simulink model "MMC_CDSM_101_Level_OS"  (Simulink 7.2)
settings: Solver=ode3  StartTime=0.0  StopTime=0.25  FixedStep=4e-6  MaxStep=5e-5  RelTol=1e-3  AbsTol=1e-3
PreLoadFcn:
  | INIT_MMC_100L
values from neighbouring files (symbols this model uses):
  C = 5e-3*1    (= 0.005)    [INIT_MMC_100L.m]    (also in INIT_MMC_200L.m; INIT_MMC_20L.m = 0.01; INIT_MMC_400L.m = 0.01; INIT_B6_2L_3Ph_IGBT_OS.m = 0.01)
  F = 50    [INIT_MMC_100L.m]    (also in INIT_MMC_200L.m; INIT_MMC_20L.m; INIT_MMC_400L.m; INIT_B6_2L_3Ph_IGBT_OS.m)
  FS = 50    [INIT_MMC_100L.m]    (also in INIT_MMC_200L.m; INIT_MMC_20L.m = 150; INIT_MMC_400L.m; INIT_B6_2L_3Ph_IGBT_OS.m = 900)
  I_B = INS    [INIT_MMC_100L.m]    (also in INIT_MMC_200L.m; INIT_MMC_20L.m; INIT_MMC_400L.m; INIT_B6_2L_3Ph_IGBT_OS.m)
  IDC = PDC/VDC    (= 1562.5)    [INIT_MMC_100L.m]    (also in INIT_MMC_200L.m; INIT_MMC_20L.m = 1000; INIT_MMC_400L.m; INIT_B6_2L_3Ph_IGBT_OS.m = 166.666666667)
  KI2 = 0.01    [INIT_MMC_100L.m]    (also in INIT_MMC_200L.m = 100; INIT_MMC_20L.m = 0.1; INIT_MMC_400L.m = 0.1)
  KP2 = 0.2    [INIT_MMC_100L.m]    (also in INIT_MMC_200L.m; INIT_MMC_20L.m = 1; INIT_MMC_400L.m)
  LN = 25e-3    (= 0.025)    [INIT_MMC_100L.m]    (also in INIT_MMC_200L.m; INIT_MMC_20L.m = 0.002; INIT_MMC_400L.m; INIT_PWM_2L.m = 0.002)
  LNpu = LN/L_B    [INIT_MMC_100L.m]    (also in INIT_MMC_200L.m; INIT_MMC_20L.m; INIT_MMC_400L.m; INIT_PWM_2L.m)
  LS = 25e-3    (= 0.025)    [INIT_MMC_100L.m]    (also in INIT_MMC_200L.m; INIT_MMC_20L.m = 0.0025; INIT_MMC_400L.m; INIT_B6_2L_3Ph_IGBT_OS.m = 0.001)
  LSpu = LS/L_B    [INIT_MMC_100L.m]    (also in INIT_MMC_200L.m; INIT_MMC_20L.m; INIT_MMC_400L.m; INIT_B6_2L_3Ph_IGBT_OS.m)
  LT = LN    (= 0.025)    [INIT_MMC_100L.m]    (also in INIT_MMC_200L.m; INIT_MMC_20L.m = 0.002; INIT_MMC_400L.m)
  Nc = 100    [INIT_MMC_100L.m]    (also in INIT_MMC_200L.m = 200; INIT_MMC_20L.m = 20; INIT_MMC_400L.m = 400)
  NT = sqrt(3)*340/400    [INIT_MMC_100L.m]    (also in INIT_MMC_200L.m; INIT_MMC_20L.m = sqrt(3); INIT_MMC_400L.m)
  RN = 0.1    [INIT_MMC_100L.m]    (also in INIT_MMC_200L.m; INIT_MMC_20L.m; INIT_MMC_400L.m; INIT_PWM_2L.m)
  RT = RN    (= 0.1)    [INIT_MMC_100L.m]    (also in INIT_MMC_200L.m; INIT_MMC_20L.m; INIT_MMC_400L.m)
  U_B = UNS    [INIT_MMC_100L.m]    (also in INIT_MMC_200L.m; INIT_MMC_20L.m; INIT_MMC_400L.m; INIT_B6_2L_3Ph_IGBT_OS.m)
  UC0 = 3.4e3*2    (= 6800)    [INIT_MMC_100L.m]    (also in INIT_MMC_200L.m = 3400; INIT_MMC_20L.m = 5000; INIT_MMC_400L.m = 1700; INIT_B6_2L_3Ph_IGBT_OS.m = 600)
  UNP = ULLP/sqrt(3)    [INIT_MMC_100L.m]    (also in INIT_MMC_200L.m; INIT_MMC_20L.m; INIT_MMC_400L.m; INIT_B6_2L_3Ph_IGBT_OS.m)
  UNS = ULLP/sqrt(3)*340/400    [INIT_MMC_100L.m]    (also in INIT_MMC_200L.m; INIT_MMC_20L.m = ULLP/sqrt(3); INIT_MMC_400L.m; INIT_B6_2L_3Ph_IGBT_OS.m = ULLP/sqrt(3))
  VDC = 640e3    (= 640000)    [INIT_MMC_100L.m]    (also in INIT_MMC_200L.m; INIT_MMC_20L.m = 100000; INIT_MMC_400L.m; INIT_B6_2L_3Ph_IGBT_OS.m = 600)
libraries: simulink x1

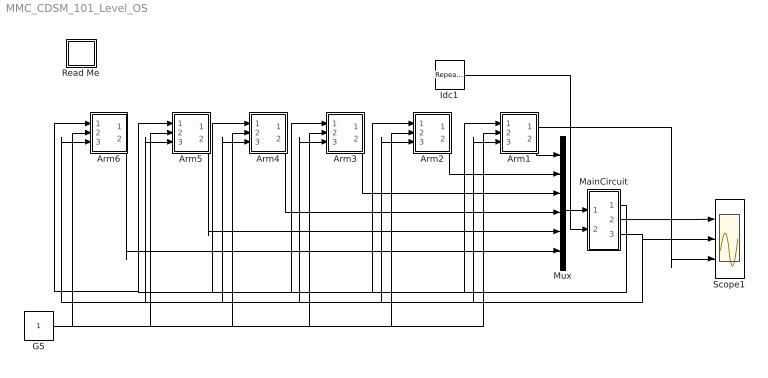
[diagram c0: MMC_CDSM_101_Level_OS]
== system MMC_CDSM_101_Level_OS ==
  Arm1 : Subsystem
  Arm2 : Subsystem
  Arm3 : Subsystem
  Arm4 : Subsystem
  Arm5 : Subsystem
  Arm6 : Subsystem
  G5 : Constant  OutDataType=sfix(16)  OutScaling=2^0
  Idc1 : simulink/Sources/Repeating Sequence  SystemSampleTime=-1  rep_seq_t="[0    0.1   0.101   0.15    0.151   5 ]"  rep_seq_y="[1     1       0.0        0.0       -1         -1 ]*IDC"
  MainCircuit : Subsystem
  Mux : Mux  Inputs=6
  Read Me : Subsystem
  Scope1 : Scope  NumInputPorts=3
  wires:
  Mux/1 -> MainCircuit/1(V)
  MainCircuit/1(G) -> Arm1/1(G1), Arm5/1(G1), Arm6/1(G1), Arm4/1(G1), Arm3/1(G1), Arm2/1(G1)
  MainCircuit/3(ILs) -> Arm1/3(ILs), Arm5/3(ILs), Arm6/3(ILs), Arm4/3(ILs), Arm3/3(ILs), Arm2/3(ILs), Scope1/2
  Idc1/1 -> MainCircuit/2(Idc)
  MainCircuit/2(IWR) -> Scope1/1
  Arm1/1(VC) -> Scope1/3
  Arm1/2(V1) -> Mux/1
  Arm2/2(V1) -> Mux/2
  Arm3/2(V1) -> Mux/3
  Arm4/2(V1) -> Mux/4
  Arm5/2(V1) -> Mux/5
  Arm6/2(V1) -> Mux/6
  G5/1 -> Arm1/2(G5), Arm2/2(G5), Arm3/2(G5), Arm4/2(G5), Arm5/2(G5), Arm6/2(G5)

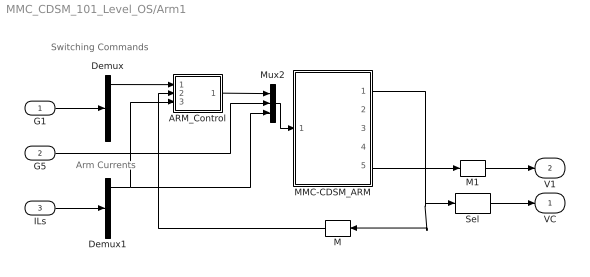
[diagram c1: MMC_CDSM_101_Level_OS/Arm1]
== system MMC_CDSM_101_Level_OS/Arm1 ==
  note: Switching Commands
  note: Arm Currents
  G1 : Inport
  G5 : Inport  Port=2
  ILs : Inport  Port=3
  ARM_Control : Subsystem
  Demux : Demux  Outputs=6
  Demux1 : Demux  Outputs=6
  M : Memory  Orientation=left
  M1 : Memory
  MMC-CDSM_ARM : Subsystem  mask(MMC_HB_ARM){C=C, UC0=UC0, Nc=Nc}
      mask prompts: C "C [F]"; UC0 "UC0 [V]"; Nc "Number Caps"
      mask help: Input Vector Switching Signals Arm Current Output Vector Capacitor Voltages Capacitor Current IT1, ID1, VT1, IT2, ID2, VT2 Arm Voltage Parameter Vector Capacitor Value =p[0] Initial Capacitor Voltage =p[1] Number of Cap. =p[2]
  Mux2 : Mux  Inputs="[2*Nc  1  1]"
  Sel : Selector  InputPortWidth=Nc  IndexOptions=Index vector (dialog)  Indices=[1 2 3 4 5 6 7 8 9 10]  OutputSizes=1
  VC : Outport
  V1 : Outport  Port=2
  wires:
  ARM_Control/1(O1) -> Mux2/1
  ILs/1 -> Demux1/1
  MMC-CDSM_ARM/1(VCs) -> M/1, Sel/1
  M/1 -> ARM_Control/2(Uc)
  Demux1/1 -> ARM_Control/3(ILs), Mux2/3
  G1/1 -> Demux/1
  Demux/1 -> ARM_Control/1(S)
  Mux2/1 -> MMC-CDSM_ARM/1(In)
  MMC-CDSM_ARM/5(V_arm) -> M1/1
  M1/1 -> V1/1
  Sel/1 -> VC/1
  G5/1 -> Mux2/2

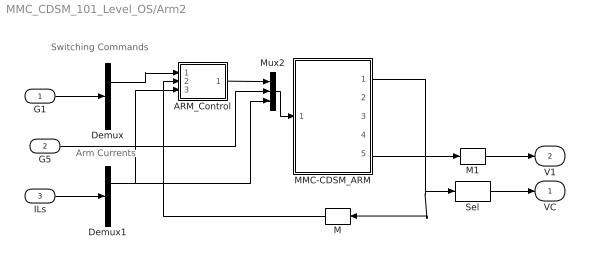
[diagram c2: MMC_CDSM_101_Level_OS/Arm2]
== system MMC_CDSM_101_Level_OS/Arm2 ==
  note: Arm Currents
  note: Switching Commands
  G1 : Inport
  G5 : Inport  Port=2
  ILs : Inport  Port=3
  ARM_Control : Subsystem
  Demux : Demux  Outputs=6
  Demux1 : Demux  Outputs=6
  M : Memory  Orientation=left
  M1 : Memory
  MMC-CDSM_ARM : Subsystem  mask(MMC_HB_ARM){C=C, UC0=UC0, Nc=Nc}
      mask prompts: C "C [F]"; UC0 "UC0 [V]"; Nc "Number Caps"
      mask help: Input Vector Switching Signals Arm Current Output Vector Capacitor Voltages Capacitor Current IT1, ID1, VT1, IT2, ID2, VT2 Arm Voltage Parameter Vector Capacitor Value =p[0] Initial Capacitor Voltage =p[1] Number of Cap. =p[2]
  Mux2 : Mux  Inputs="[2*Nc 1  1]"
  Sel : Selector  InputPortWidth=Nc  IndexOptions=Index vector (dialog)  Indices=[1 2 3 4 5 6 7 8 9 10]  OutputSizes=1
  VC : Outport
  V1 : Outport  Port=2
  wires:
  Sel/1 -> VC/1
  M1/1 -> V1/1
  MMC-CDSM_ARM/5(V_arm) -> M1/1
  Mux2/1 -> MMC-CDSM_ARM/1(In)
  G1/1 -> Demux/1
  M/1 -> ARM_Control/2(Uc)
  MMC-CDSM_ARM/1(VCs) -> Sel/1, M/1
  ILs/1 -> Demux1/1
  ARM_Control/1(O1) -> Mux2/1
  Demux1/2 -> ARM_Control/3(ILs), Mux2/3
  Demux/2 -> ARM_Control/1(S)
  G5/1 -> Mux2/2

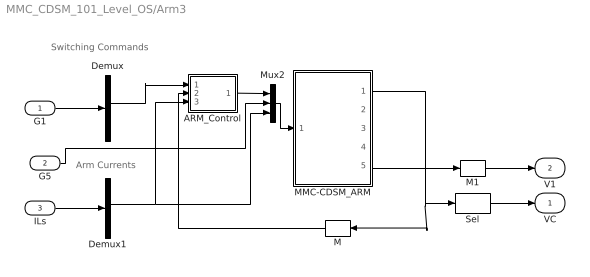
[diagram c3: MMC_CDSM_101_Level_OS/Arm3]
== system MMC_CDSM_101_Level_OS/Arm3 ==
  note: Switching Commands
  note: Arm Currents
  G1 : Inport
  G5 : Inport  Port=2
  ILs : Inport  Port=3
  ARM_Control : Subsystem
  Demux : Demux  Outputs=6
  Demux1 : Demux  Outputs=6
  M : Memory  Orientation=left
  M1 : Memory
  MMC-CDSM_ARM : Subsystem  mask(MMC_HB_ARM){C=C, UC0=UC0, Nc=Nc}
      mask prompts: C "C [F]"; UC0 "UC0 [V]"; Nc "Number Caps"
      mask help: Input Vector Switching Signals Arm Current Output Vector Capacitor Voltages Capacitor Current IT1, ID1, VT1, IT2, ID2, VT2 Arm Voltage Parameter Vector Capacitor Value =p[0] Initial Capacitor Voltage =p[1] Number of Cap. =p[2]
  Mux2 : Mux  Inputs="[2*Nc  1  1]"
  Sel : Selector  InputPortWidth=Nc  IndexOptions=Index vector (dialog)  Indices=[1 2 3 4 5 6 7 8 9 10]  OutputSizes=1
  VC : Outport
  V1 : Outport  Port=2
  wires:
  ARM_Control/1(O1) -> Mux2/1
  ILs/1 -> Demux1/1
  MMC-CDSM_ARM/1(VCs) -> M/1, Sel/1
  M/1 -> ARM_Control/2(Uc)
  G1/1 -> Demux/1
  Mux2/1 -> MMC-CDSM_ARM/1(In)
  MMC-CDSM_ARM/5(V_arm) -> M1/1
  M1/1 -> V1/1
  Sel/1 -> VC/1
  Demux1/3 -> ARM_Control/3(ILs), Mux2/3
  Demux/3 -> ARM_Control/1(S)
  G5/1 -> Mux2/2

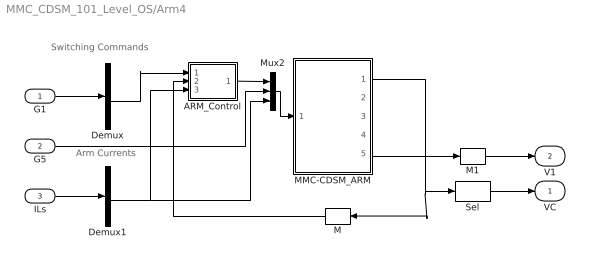
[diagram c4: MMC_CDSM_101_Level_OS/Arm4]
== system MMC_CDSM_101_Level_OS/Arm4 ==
  note: Arm Currents
  note: Switching Commands
  G1 : Inport
  G5 : Inport  Port=2
  ILs : Inport  Port=3
  ARM_Control : Subsystem
  Demux : Demux  Outputs=6
  Demux1 : Demux  Outputs=6
  M : Memory  Orientation=left
  M1 : Memory
  MMC-CDSM_ARM : Subsystem  mask(MMC_HB_ARM){C=C, UC0=UC0, Nc=Nc}
      mask prompts: C "C [F]"; UC0 "UC0 [V]"; Nc "Number Caps"
      mask help: Input Vector Switching Signals Arm Current Output Vector Capacitor Voltages Capacitor Current IT1, ID1, VT1, IT2, ID2, VT2 Arm Voltage Parameter Vector Capacitor Value =p[0] Initial Capacitor Voltage =p[1] Number of Cap. =p[2]
  Mux2 : Mux  Inputs="[2*Nc  1  1]"
  Sel : Selector  InputPortWidth=Nc  IndexOptions=Index vector (dialog)  Indices=[1 2 3 4 5 6 7 8 9 10]  OutputSizes=1
  VC : Outport
  V1 : Outport  Port=2
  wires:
  Sel/1 -> VC/1
  M1/1 -> V1/1
  MMC-CDSM_ARM/5(V_arm) -> M1/1
  Mux2/1 -> MMC-CDSM_ARM/1(In)
  G1/1 -> Demux/1
  M/1 -> ARM_Control/2(Uc)
  MMC-CDSM_ARM/1(VCs) -> Sel/1, M/1
  ILs/1 -> Demux1/1
  ARM_Control/1(O1) -> Mux2/1
  Demux1/4 -> ARM_Control/3(ILs), Mux2/3
  Demux/4 -> ARM_Control/1(S)
  G5/1 -> Mux2/2

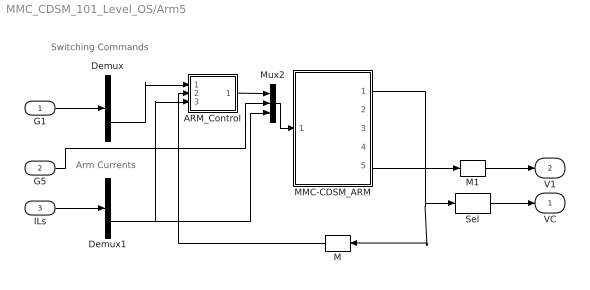
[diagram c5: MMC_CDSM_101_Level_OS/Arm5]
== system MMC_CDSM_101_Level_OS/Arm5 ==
  note: Switching Commands
  note: Arm Currents
  G1 : Inport
  G5 : Inport  Port=2
  ILs : Inport  Port=3
  ARM_Control : Subsystem
  Demux : Demux  Outputs=6
  Demux1 : Demux  Outputs=6
  M : Memory  Orientation=left
  M1 : Memory
  MMC-CDSM_ARM : Subsystem  mask(MMC_HB_ARM){C=C, UC0=UC0, Nc=Nc}
      mask prompts: C "C [F]"; UC0 "UC0 [V]"; Nc "Number Caps"
      mask help: Input Vector Switching Signals Arm Current Output Vector Capacitor Voltages Capacitor Current IT1, ID1, VT1, IT2, ID2, VT2 Arm Voltage Parameter Vector Capacitor Value =p[0] Initial Capacitor Voltage =p[1] Number of Cap. =p[2]
  Mux2 : Mux  Inputs="[2*Nc  1   1]"
  Sel : Selector  InputPortWidth=Nc  IndexOptions=Index vector (dialog)  Indices=[1 2 3 4 5 6 7 8 9 10]  OutputSizes=1
  VC : Outport
  V1 : Outport  Port=2
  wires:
  ARM_Control/1(O1) -> Mux2/1
  ILs/1 -> Demux1/1
  MMC-CDSM_ARM/1(VCs) -> M/1, Sel/1
  M/1 -> ARM_Control/2(Uc)
  G1/1 -> Demux/1
  Mux2/1 -> MMC-CDSM_ARM/1(In)
  MMC-CDSM_ARM/5(V_arm) -> M1/1
  M1/1 -> V1/1
  Sel/1 -> VC/1
  Demux1/5 -> ARM_Control/3(ILs), Mux2/3
  Demux/5 -> ARM_Control/1(S)
  G5/1 -> Mux2/2

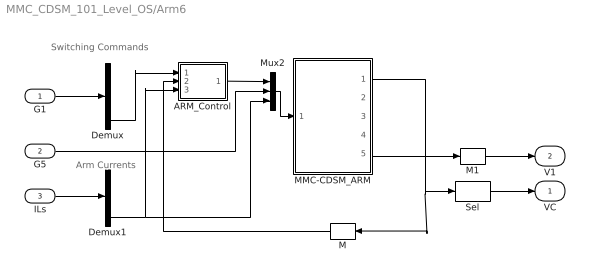
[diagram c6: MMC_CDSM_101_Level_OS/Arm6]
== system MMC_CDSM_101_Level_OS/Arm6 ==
  note: Arm Currents
  note: Switching Commands
  G1 : Inport
  G5 : Inport  Port=2
  ILs : Inport  Port=3
  ARM_Control : Subsystem
  Demux : Demux  Outputs=6
  Demux1 : Demux  Outputs=6
  M : Memory  Orientation=left
  M1 : Memory
  MMC-CDSM_ARM : Subsystem  mask(MMC_HB_ARM){C=C, UC0=UC0, Nc=Nc}
      mask prompts: C "C [F]"; UC0 "UC0 [V]"; Nc "Number Caps"
      mask help: Input Vector Switching Signals Arm Current Output Vector Capacitor Voltages Capacitor Current IT1, ID1, VT1, IT2, ID2, VT2 Arm Voltage Parameter Vector Capacitor Value =p[0] Initial Capacitor Voltage =p[1] Number of Cap. =p[2]
  Mux2 : Mux  Inputs="[2*Nc  1  1]"
  Sel : Selector  InputPortWidth=Nc  IndexOptions=Index vector (dialog)  Indices=[1 2 3 4 5 6 7 8 9 10]  OutputSizes=1
  VC : Outport
  V1 : Outport  Port=2
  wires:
  Sel/1 -> VC/1
  M1/1 -> V1/1
  MMC-CDSM_ARM/5(V_arm) -> M1/1
  Mux2/1 -> MMC-CDSM_ARM/1(In)
  G1/1 -> Demux/1
  M/1 -> ARM_Control/2(Uc)
  MMC-CDSM_ARM/1(VCs) -> Sel/1, M/1
  ILs/1 -> Demux1/1
  ARM_Control/1(O1) -> Mux2/1
  Demux1/6 -> ARM_Control/3(ILs), Mux2/3
  Demux/6 -> ARM_Control/1(S)
  G5/1 -> Mux2/2

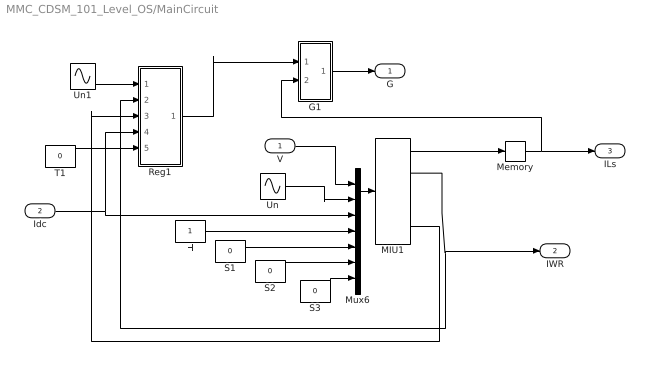
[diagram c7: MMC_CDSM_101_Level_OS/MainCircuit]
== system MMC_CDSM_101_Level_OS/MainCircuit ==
  V : Inport
  Idc : Inport  Port=2
  G1 : Subsystem
  H : Constant  OutDataType=sfix(16)  OutScaling=2^0
  MIU1 : S-Function  FunctionName=s_MMC_MC_TYD_SC  Parameters="[LS LN RN LT RT  NT Rg]"  EnableBusSupport=off  mask{LS=LS*1, LN=LN*1, RN=RN*1, LT=LT, RT=RT, NT=NT, Rg=1e-3}
  Memory : Memory
  Mux6 : Mux  Inputs="[6  3  1  1   1   1    1]"
  Reg1 : Subsystem
  S1 : Constant  Value=0  OutDataType=sfix(16)  OutScaling=2^0
  S2 : Constant  Value=0  OutDataType=sfix(16)  OutScaling=2^0
  S3 : Constant  Value=0  OutDataType=sfix(16)  OutScaling=2^0
  T1 : Constant  Value=0
  Un : Sin  Amplitude=UNP*0.999  Frequency=2*pi*F  Phase="[0   -2*pi/3    -4*pi/3]"  SampleTime=0
  Un1 : Sin  Amplitude=UNS*0.999  Frequency=2*pi*F  Phase="[-pi/6*5   -2*pi/3-pi/6*5     -4*pi/3-pi/6*5 ]"  SampleTime=0
  G : Outport
  IWR : Outport  Port=2
  ILs : Outport  Port=3
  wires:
  Idc/1 -> Mux6/3, Reg1/4(Id*)
  MIU1/2 -> IWR/1, Reg1/2(Iwr)
  Memory/1 -> ILs/1, G1/2(ILs)
  G1/1(S) -> G/1
  Mux6/1 -> MIU1/1
  MIU1/1 -> Memory/1
  Reg1/1(A) -> G1/1(A)
  T1/1 -> Reg1/5(Iq1*)
  MIU1/5 -> Reg1/3(UDC)
  Un1/1 -> Reg1/1(UN)
  V/1 -> Mux6/1
  Un/1 -> Mux6/2
  H/1 -> Mux6/4
  S1/1 -> Mux6/5
  S2/1 -> Mux6/6
  S3/1 -> Mux6/7

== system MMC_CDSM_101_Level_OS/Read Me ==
  note: MMC 101 Level CDSM-Converter using circuit partitioning
  note: The model demonstrate the modeling of the CDSM bridge 101-Level 3-phase MMC-Converter using Circuit Partitioning. The converter arm is modeled as one CDSM bridge 100-Level Subcircuit. The converter is operating in 3 modes: from 0-0.1 sec in Motoring mode from 0.1-0.15 sec no load mode from 0.15- 0.25 sec in generating mode Scope1: 3 Phase MMC-Converter Currents 6 Arm-Inductor currents 10 Capacitor Voltages Using Fixed Step 20 micro seconds, Solver ode3(Bogacki-Shampine) on my intel(R) Core(TM) i9-10900K CPU, 3,7 GHz we get: S-Function NAME = MMC_MC_TYD_SC System Matrix Dimentions = 51 * 51 S-Function NAME = MMC_CDSM_ARM System Matrix Dimentions = 250 * 250 Elapsed time is 5.053354 seconds

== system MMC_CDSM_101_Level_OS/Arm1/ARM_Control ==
  S : Inport
  Uc : Inport  Port=2
  ILs : Inport  Port=3
  Mux : Mux  Inputs="[Nc Nc  1]"
  SELECT_C : S-Function  FunctionName=SELECT_MMC_C  Parameters=2*Nc  EnableBusSupport=off
  O1 : Outport
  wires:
  ILs/1 -> Mux/3
  SELECT_C/1 -> O1/1
  Mux/1 -> SELECT_C/1
  S/1 -> Mux/1
  Uc/1 -> Mux/2

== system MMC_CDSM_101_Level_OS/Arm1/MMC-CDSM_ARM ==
  In : Inport  OutDataType=sfix(16)  OutScaling=2^0
  MMC_CDSM_ARM : S-Function  FunctionName=s_MMC_CDSM_ARM  Parameters="[C   UC0   Nc]"  EnableBusSupport=off
  VCs : Outport  OutDataType=sfix(16)  OutScaling=2^0
  IC1 : Outport  Port=2  OutDataType=sfix(16)  OutScaling=2^0
  IT1,ID1,VT1 : Outport  Port=3  OutDataType=sfix(16)  OutScaling=2^0
  IT2,ID2,VT2 : Outport  Port=4  OutDataType=sfix(16)  OutScaling=2^0
  V_arm : Outport  Port=5  OutDataType=sfix(16)  OutScaling=2^0
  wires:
  In/1 -> MMC_CDSM_ARM/1
  MMC_CDSM_ARM/1 -> VCs/1
  MMC_CDSM_ARM/2 -> IC1/1
  MMC_CDSM_ARM/3 -> IT1,ID1,VT1/1
  MMC_CDSM_ARM/4 -> IT2,ID2,VT2/1
  MMC_CDSM_ARM/5 -> V_arm/1

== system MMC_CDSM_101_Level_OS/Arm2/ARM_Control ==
  S : Inport
  Uc : Inport  Port=2
  ILs : Inport  Port=3
  Mux : Mux  Inputs="[Nc Nc  1]"
  SELECT_C : S-Function  FunctionName=SELECT_MMC_C  Parameters=2*Nc  EnableBusSupport=off
  O1 : Outport
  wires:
  Uc/1 -> Mux/2
  S/1 -> Mux/1
  Mux/1 -> SELECT_C/1
  SELECT_C/1 -> O1/1
  ILs/1 -> Mux/3

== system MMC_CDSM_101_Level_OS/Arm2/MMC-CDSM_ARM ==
  In : Inport  OutDataType=sfix(16)  OutScaling=2^0
  MMC_CDSM_ARM : S-Function  FunctionName=s_MMC_CDSM_ARM  Parameters="[C   UC0   Nc]"  EnableBusSupport=off
  VCs : Outport  OutDataType=sfix(16)  OutScaling=2^0
  IC1 : Outport  Port=2  OutDataType=sfix(16)  OutScaling=2^0
  IT1,ID1,VT1 : Outport  Port=3  OutDataType=sfix(16)  OutScaling=2^0
  IT2,ID2,VT2 : Outport  Port=4  OutDataType=sfix(16)  OutScaling=2^0
  V_arm : Outport  Port=5  OutDataType=sfix(16)  OutScaling=2^0
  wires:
  MMC_CDSM_ARM/5 -> V_arm/1
  MMC_CDSM_ARM/4 -> IT2,ID2,VT2/1
  MMC_CDSM_ARM/3 -> IT1,ID1,VT1/1
  MMC_CDSM_ARM/2 -> IC1/1
  MMC_CDSM_ARM/1 -> VCs/1
  In/1 -> MMC_CDSM_ARM/1

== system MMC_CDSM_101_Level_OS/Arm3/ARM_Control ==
  S : Inport
  Uc : Inport  Port=2
  ILs : Inport  Port=3
  Mux : Mux  Inputs="[Nc Nc  1]"
  SELECT_C : S-Function  FunctionName=SELECT_MMC_C  Parameters=2*Nc  EnableBusSupport=off
  O1 : Outport
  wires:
  ILs/1 -> Mux/3
  SELECT_C/1 -> O1/1
  Mux/1 -> SELECT_C/1
  S/1 -> Mux/1
  Uc/1 -> Mux/2

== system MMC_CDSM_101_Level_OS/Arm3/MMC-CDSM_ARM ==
  In : Inport  OutDataType=sfix(16)  OutScaling=2^0
  MMC_CDSM_ARM : S-Function  FunctionName=s_MMC_CDSM_ARM  Parameters="[C   UC0   Nc]"  EnableBusSupport=off
  VCs : Outport  OutDataType=sfix(16)  OutScaling=2^0
  IC1 : Outport  Port=2  OutDataType=sfix(16)  OutScaling=2^0
  IT1,ID1,VT1 : Outport  Port=3  OutDataType=sfix(16)  OutScaling=2^0
  IT2,ID2,VT2 : Outport  Port=4  OutDataType=sfix(16)  OutScaling=2^0
  V_arm : Outport  Port=5  OutDataType=sfix(16)  OutScaling=2^0
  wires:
  In/1 -> MMC_CDSM_ARM/1
  MMC_CDSM_ARM/1 -> VCs/1
  MMC_CDSM_ARM/2 -> IC1/1
  MMC_CDSM_ARM/3 -> IT1,ID1,VT1/1
  MMC_CDSM_ARM/4 -> IT2,ID2,VT2/1
  MMC_CDSM_ARM/5 -> V_arm/1

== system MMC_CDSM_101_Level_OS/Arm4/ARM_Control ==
  S : Inport
  Uc : Inport  Port=2
  ILs : Inport  Port=3
  Mux : Mux  Inputs="[Nc Nc  1]"
  SELECT_C : S-Function  FunctionName=SELECT_MMC_C  Parameters=2*Nc  EnableBusSupport=off
  O1 : Outport
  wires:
  Uc/1 -> Mux/2
  S/1 -> Mux/1
  Mux/1 -> SELECT_C/1
  SELECT_C/1 -> O1/1
  ILs/1 -> Mux/3

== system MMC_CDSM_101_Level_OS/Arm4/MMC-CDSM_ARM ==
  In : Inport  OutDataType=sfix(16)  OutScaling=2^0
  MMC_CDSM_ARM : S-Function  FunctionName=s_MMC_CDSM_ARM  Parameters="[C   UC0   Nc]"  EnableBusSupport=off
  VCs : Outport  OutDataType=sfix(16)  OutScaling=2^0
  IC1 : Outport  Port=2  OutDataType=sfix(16)  OutScaling=2^0
  IT1,ID1,VT1 : Outport  Port=3  OutDataType=sfix(16)  OutScaling=2^0
  IT2,ID2,VT2 : Outport  Port=4  OutDataType=sfix(16)  OutScaling=2^0
  V_arm : Outport  Port=5  OutDataType=sfix(16)  OutScaling=2^0
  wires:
  MMC_CDSM_ARM/5 -> V_arm/1
  MMC_CDSM_ARM/4 -> IT2,ID2,VT2/1
  MMC_CDSM_ARM/3 -> IT1,ID1,VT1/1
  MMC_CDSM_ARM/2 -> IC1/1
  MMC_CDSM_ARM/1 -> VCs/1
  In/1 -> MMC_CDSM_ARM/1

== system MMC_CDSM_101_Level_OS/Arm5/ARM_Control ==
  S : Inport
  Uc : Inport  Port=2
  ILs : Inport  Port=3
  Mux : Mux  Inputs="[Nc Nc  1]"
  SELECT_C : S-Function  FunctionName=SELECT_MMC_C  Parameters=2*Nc  EnableBusSupport=off
  O1 : Outport
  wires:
  ILs/1 -> Mux/3
  SELECT_C/1 -> O1/1
  Mux/1 -> SELECT_C/1
  S/1 -> Mux/1
  Uc/1 -> Mux/2

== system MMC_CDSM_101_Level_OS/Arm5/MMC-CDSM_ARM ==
  In : Inport  OutDataType=sfix(16)  OutScaling=2^0
  MMC_CDSM_ARM : S-Function  FunctionName=s_MMC_CDSM_ARM  Parameters="[C   UC0   Nc]"  EnableBusSupport=off
  VCs : Outport  OutDataType=sfix(16)  OutScaling=2^0
  IC1 : Outport  Port=2  OutDataType=sfix(16)  OutScaling=2^0
  IT1,ID1,VT1 : Outport  Port=3  OutDataType=sfix(16)  OutScaling=2^0
  IT2,ID2,VT2 : Outport  Port=4  OutDataType=sfix(16)  OutScaling=2^0
  V_arm : Outport  Port=5  OutDataType=sfix(16)  OutScaling=2^0
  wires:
  In/1 -> MMC_CDSM_ARM/1
  MMC_CDSM_ARM/1 -> VCs/1
  MMC_CDSM_ARM/2 -> IC1/1
  MMC_CDSM_ARM/3 -> IT1,ID1,VT1/1
  MMC_CDSM_ARM/4 -> IT2,ID2,VT2/1
  MMC_CDSM_ARM/5 -> V_arm/1

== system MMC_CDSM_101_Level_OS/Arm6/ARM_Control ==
  S : Inport
  Uc : Inport  Port=2
  ILs : Inport  Port=3
  Mux : Mux  Inputs="[Nc Nc  1]"
  SELECT_C : S-Function  FunctionName=SELECT_MMC_C  Parameters=2*Nc  EnableBusSupport=off
  O1 : Outport
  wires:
  Uc/1 -> Mux/2
  S/1 -> Mux/1
  Mux/1 -> SELECT_C/1
  SELECT_C/1 -> O1/1
  ILs/1 -> Mux/3

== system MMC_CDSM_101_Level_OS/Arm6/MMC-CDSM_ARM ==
  In : Inport  OutDataType=sfix(16)  OutScaling=2^0
  MMC_CDSM_ARM : S-Function  FunctionName=s_MMC_CDSM_ARM  Parameters="[C   UC0   Nc]"  EnableBusSupport=off
  VCs : Outport  OutDataType=sfix(16)  OutScaling=2^0
  IC1 : Outport  Port=2  OutDataType=sfix(16)  OutScaling=2^0
  IT1,ID1,VT1 : Outport  Port=3  OutDataType=sfix(16)  OutScaling=2^0
  IT2,ID2,VT2 : Outport  Port=4  OutDataType=sfix(16)  OutScaling=2^0
  V_arm : Outport  Port=5  OutDataType=sfix(16)  OutScaling=2^0
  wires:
  MMC_CDSM_ARM/5 -> V_arm/1
  MMC_CDSM_ARM/4 -> IT2,ID2,VT2/1
  MMC_CDSM_ARM/3 -> IT1,ID1,VT1/1
  MMC_CDSM_ARM/2 -> IC1/1
  MMC_CDSM_ARM/1 -> VCs/1
  In/1 -> MMC_CDSM_ARM/1

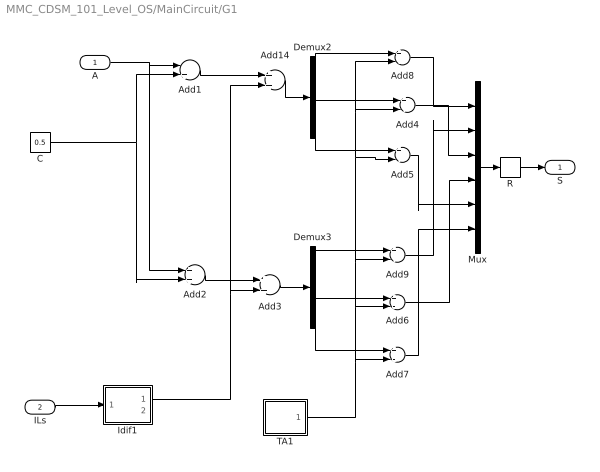
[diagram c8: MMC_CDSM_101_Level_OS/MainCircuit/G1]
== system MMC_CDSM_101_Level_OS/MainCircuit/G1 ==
  A : Inport
  ILs : Inport  Port=2
  Add1 : Sum  Inputs=-+
  Add14 : Sum
  Add2 : Sum
  Add3 : Sum
  Add{4..9} (6 alike) : Sum  Inputs=+-
  C : Constant  Value=0.5
  Demux2 : Demux  Outputs=3
  Demux3 : Demux  Outputs=3
  Idif1 : Subsystem
  Mux : Mux  Inputs=6
  R : Relay
  TA1 : Subsystem  mask(TriGtr-AO){A=0.5, O=0.5, T=1/FS, Nc=Nc}
      mask prompts: A "Amplitude"; O "Offset"; T "Period Time"; Nc "Output width"
      mask help: Triangular Wave Generator with variable time delay, variable amplitude and offset
  S : Outport
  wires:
  C/1 -> Add2/2, Add1/2
  A/1 -> Add1/1, Add2/1
  Add1/1 -> Add14/1
  Add2/1 -> Add3/1
  Idif1/1(Adiff1) -> Add3/2, Add14/2
  Add14/1 -> Demux2/1
  Demux2/1 -> Add8/1
  Demux2/2 -> Add4/1
  Demux2/3 -> Add5/1
  Mux/1 -> R/1
  Demux3/1 -> Add9/1
  Demux3/2 -> Add6/1
  Demux3/3 -> Add7/1
  Add3/1 -> Demux3/1
  TA1/1(Out1) -> Add9/2, Add8/2, Add4/2, Add5/2, Add6/2, Add7/2
  R/1 -> S/1
  ILs/1 -> Idif1/1(I1)
  Add8/1 -> Mux/1
  Add9/1 -> Mux/2
  Add4/1 -> Mux/3
  Add6/1 -> Mux/4
  Add5/1 -> Mux/5
  Add7/1 -> Mux/6

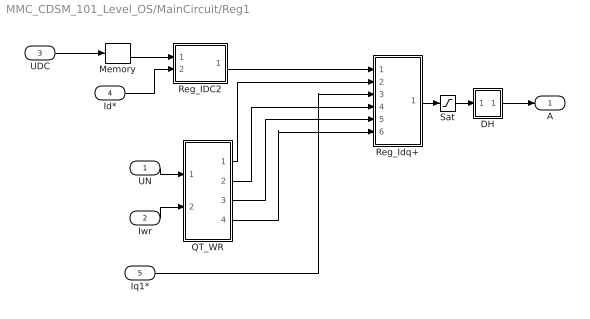
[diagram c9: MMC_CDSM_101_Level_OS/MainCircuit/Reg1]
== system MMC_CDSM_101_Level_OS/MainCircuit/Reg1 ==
  UN : Inport
  Iwr : Inport  Port=2
  UDC : Inport  Port=3
  Id* : Inport  Port=4
  Iq1* : Inport  Port=5
  DH : Subsystem
  Memory : Memory
  QT_WR : Subsystem
  Reg_IDC2 : Subsystem
  Reg_Idq+ : Subsystem
  Sat : Saturate
  A : Outport
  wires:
  QT_WR/4(Ud) -> Reg_Idq+/6(Ud)
  QT_WR/1(Id1) -> Reg_Idq+/2(Id1)
  QT_WR/2(Iq1) -> Reg_Idq+/4(Iq1)
  Iq1*/1 -> Reg_Idq+/3(Iq1*)
  QT_WR/3(th1) -> Reg_Idq+/5(th)
  Reg_IDC2/1(Id1*) -> Reg_Idq+/1(Id1*)
  Iwr/1 -> QT_WR/2(I_WR)
  UN/1 -> QT_WR/1(UN)
  UDC/1 -> Memory/1
  DH/1(O) -> A/1
  Id*/1 -> Reg_IDC2/2(Id*)
  Reg_Idq+/1(A+) -> Sat/1
  Sat/1 -> DH/1(I)
  Memory/1 -> Reg_IDC2/1(UDC)

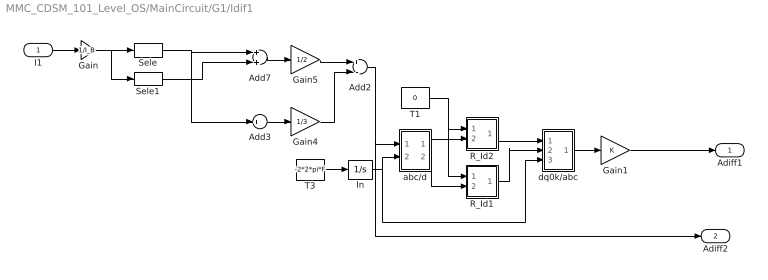
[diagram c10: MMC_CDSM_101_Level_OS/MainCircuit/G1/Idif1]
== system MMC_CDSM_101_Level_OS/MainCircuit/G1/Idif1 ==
  I1 : Inport
  Add2 : Sum  Inputs=+-
  Add3 : Sum  Inputs=+
  Add7 : Sum
  Gain : Gain  Gain=1/I_B
  Gain1 : Gain
  Gain4 : Gain  Gain=1/3
  Gain5 : Gain  Gain=1/2
  In : Integrator
  R_Id1 : Subsystem  mask(PI-controller){Kp=KP2, Ki=KI2, lim=1, Ts=-1}
      mask prompts: Kp "Proportional gain (Kp)"; Ki "Integral gain (Ki)"; lim "Output limit"; Ts "Sampling time (s)"
      mask help: Proportional-Integral Controller
  R_Id2 : Subsystem  mask(PI-controller){Kp=KP2, Ki=KI2, lim=1, Ts=-1}
      mask prompts: Kp "Proportional gain (Kp)"; Ki "Integral gain (Ki)"; lim "Output limit"; Ts "Sampling time (s)"
      mask help: Proportional-Integral Controller
  Sele : Selector  InputPortWidth=6  IndexOptions=Index vector (dialog)  Indices="[1 3  5]"  OutputSizes=1
  Sele1 : Selector  InputPortWidth=6  IndexOptions=Index vector (dialog)  Indices="[2  4  6]"  OutputSizes=1
  T1 : Constant  Value=0
  T3 : Constant  Value=-2*2*pi*F
  abc/d : Subsystem
  dq0k/abc : Subsystem
  Adiff1 : Outport
  Adiff2 : Outport  Port=2
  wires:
  T1/1 -> R_Id1/1(c*), R_Id2/1(c*)
  dq0k/abc/1(a) -> Gain1/1
  R_Id1/1(e*) -> dq0k/abc/2(qk)
  abc/d/2(qk) -> R_Id1/2(c)
  R_Id2/1(e*) -> dq0k/abc/1(dk)
  abc/d/1(dk) -> R_Id2/2(c)
  In/1 -> abc/d/2(th), dq0k/abc/3(th)
  T3/1 -> In/1
  Add2/1 -> Adiff2/1, abc/d/1(a)
  Gain4/1 -> Add2/2
  Sele1/1 -> Add7/2
  Sele/1 -> Add7/1, Add3/1
  I1/1 -> Gain/1
  Gain/1 -> Sele1/1, Sele/1
  Gain5/1 -> Add2/1
  Add7/1 -> Gain5/1
  Add3/1 -> Gain4/1
  Gain1/1 -> Adiff1/1

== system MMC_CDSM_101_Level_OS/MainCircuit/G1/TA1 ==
  Ampl. : Gain  Gain=A
  Offset : Constant  Value=O
  Sum : Sum
  TG : S-Function  FunctionName=TG_MMC  Parameters=[Nc, T]  EnableBusSupport=off
  Out1 : Outport
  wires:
  TG/1 -> Ampl./1
  Sum/1 -> Out1/1
  Ampl./1 -> Sum/1
  Offset/1 -> Sum/2

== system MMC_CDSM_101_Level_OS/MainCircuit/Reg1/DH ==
  I : Inport
  Gain : Gain  Gain=0.5
  MinMax : MinMax
  MinMax1 : MinMax  Function=max
  Sum6 : Sum  Inputs=--
  Sum7 : Sum
  O : Outport  InitialOutput=0
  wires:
  Sum7/1 -> O/1
  Gain/1 -> Sum7/2
  Sum6/1 -> Gain/1
  MinMax1/1 -> Sum6/2
  MinMax/1 -> Sum6/1
  I/1 -> Sum7/1, MinMax/1, MinMax1/1

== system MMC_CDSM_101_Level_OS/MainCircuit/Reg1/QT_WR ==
  UN : Inport
  I_WR : Inport  Port=2
  G1 : Gain  Gain=1/I_B
  Gain6 : Gain  Gain=1/U_B
  abc/dq0k1 : Subsystem
  abc/dq0k2 : Subsystem
  th3 : Subsystem
  Id1 : Outport
  Iq1 : Outport  Port=2
  th1 : Outport  Port=3
  Ud : Outport  Port=4
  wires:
  abc/dq0k1/1(dk) -> Ud/1
  abc/dq0k2/2(qk) -> Iq1/1
  abc/dq0k2/1(dk) -> Id1/1
  Gain6/1 -> abc/dq0k1/1(a), th3/1(abc)
  UN/1 -> Gain6/1
  G1/1 -> abc/dq0k2/1(a)
  I_WR/1 -> G1/1
  th3/2(th) -> abc/dq0k1/2(th), th1/1, abc/dq0k2/2(th)

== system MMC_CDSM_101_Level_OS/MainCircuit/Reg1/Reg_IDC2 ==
  UDC : Inport
  Id* : Inport  Port=2
  Add : Sum
  G1 : Gain  Gain=1/IDC
  G4 : Gain  Gain=1/VDC
  PIC : Subsystem  mask(PI-controller){Kp=5, Ki=100, lim=2, Ts=-1}
      mask prompts: Kp "Proportional gain (Kp)"; Ki "Integral gain (Ki)"; lim "Output limit"; Ts "Sampling time (s)"
      mask help: Proportional-Integral Controller
  Sat : Saturate  UpperLimit=2  LowerLimit=-2
  UDC* : Constant  Value=1.0
  Id1* : Outport
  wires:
  UDC/1 -> G4/1
  UDC*/1 -> PIC/1(c*)
  G4/1 -> PIC/2(c)
  Add/1 -> Sat/1
  Sat/1 -> Id1*/1
  PIC/1(e*) -> Add/2
  Id*/1 -> G1/1
  G1/1 -> Add/1

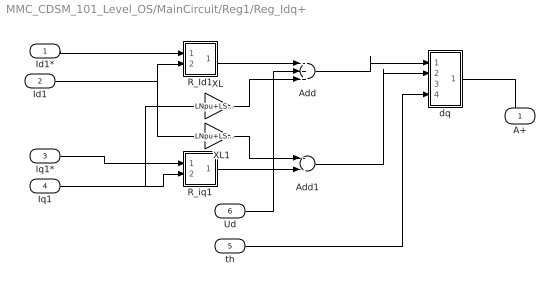
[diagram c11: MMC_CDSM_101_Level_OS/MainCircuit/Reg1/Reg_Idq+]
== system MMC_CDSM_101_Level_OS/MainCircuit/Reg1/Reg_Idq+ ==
  Id1* : Inport
  Id1 : Inport  Port=2
  Iq1* : Inport  Port=3
  Iq1 : Inport  Port=4
  th : Inport  Port=5
  Ud : Inport  Port=6
  Add : Sum  Inputs=-++
  Add1 : Sum  Inputs=--
  R_Id1 : Subsystem  mask(PI-controller){Kp=0.1, Ki=200, lim=2, Ts=-1}
      mask prompts: Kp "Proportional gain (Kp)"; Ki "Integral gain (Ki)"; lim "Output limit"; Ts "Sampling time (s)"
      mask help: Proportional-Integral Controller
  R_iq1 : Subsystem  mask(PI-controller){Kp=0.1, Ki=200, lim=2, Ts=-2}
      mask prompts: Kp "Proportional gain (Kp)"; Ki "Integral gain (Ki)"; lim "Output limit"; Ts "Sampling time (s)"
      mask help: Proportional-Integral Controller
  XL : Gain  Gain=LNpu+LSpu/2
  XL1 : Gain  Gain=LNpu+LSpu/2
  dq : Subsystem
  A+ : Outport
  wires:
  Add1/1 -> dq/2(qk)
  Add/1 -> dq/1(dk)
  R_iq1/1(e*) -> Add1/2
  Ud/1 -> Add/2
  R_Id1/1(e*) -> Add/1
  th/1 -> dq/4(th)
  dq/1(a) -> A+/1
  Id1*/1 -> R_Id1/1(c*)
  Id1/1 -> XL1/1, R_Id1/2(c)
  Iq1*/1 -> R_iq1/1(c*)
  Iq1/1 -> XL/1, R_iq1/2(c)
  XL/1 -> Add/3
  XL1/1 -> Add1/1

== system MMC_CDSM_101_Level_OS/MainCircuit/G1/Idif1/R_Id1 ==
  c* : Inport
  c : Inport  Port=2
  Gain : Gain  Gain=Ki
  Gain1 : Gain  Gain=Kp
  Integrator : Integrator  UpperSaturationLimit=lim  LowerSaturationLimit=-lim
  Saturation : Saturate  UpperLimit=lim  LowerLimit=-lim
  Sum1 : Sum  Inputs=+-
  Sum2 : Sum
  e* : Outport  InitialOutput=0
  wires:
  Gain/1 -> Integrator/1
  Gain1/1 -> Sum2/1
  Sum1/1 -> Gain/1, Gain1/1
  Sum2/1 -> Saturation/1
  Saturation/1 -> e*/1
  c/1 -> Sum1/2
  c*/1 -> Sum1/1
  Integrator/1 -> Sum2/2

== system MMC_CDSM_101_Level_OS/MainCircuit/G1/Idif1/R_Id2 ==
  c* : Inport
  c : Inport  Port=2
  Gain : Gain  Gain=Ki
  Gain1 : Gain  Gain=Kp
  Integrator : Integrator  UpperSaturationLimit=lim  LowerSaturationLimit=-lim
  Saturation : Saturate  UpperLimit=lim  LowerLimit=-lim
  Sum1 : Sum  Inputs=+-
  Sum2 : Sum
  e* : Outport  InitialOutput=0
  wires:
  Integrator/1 -> Sum2/2
  c*/1 -> Sum1/1
  c/1 -> Sum1/2
  Saturation/1 -> e*/1
  Sum2/1 -> Saturation/1
  Sum1/1 -> Gain1/1, Gain/1
  Gain1/1 -> Sum2/1
  Gain/1 -> Integrator/1

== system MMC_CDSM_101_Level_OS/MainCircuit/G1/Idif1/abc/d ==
  a : Inport
  th : Inport  Port=2
  Demux : Demux  Outputs=3
  Fcn : Fcn  Expr=u(1)*cos(u(3)) + u(2)*sin(u(3))
  Fcn1 : Fcn  Expr=-u(1)*sin(u(3)) + u(2)*cos(u(3))
  K : Gain  Gain="2/3*[1   -.5   -.5;  0   sqrt(3)/2   -sqrt(3)/2;  .5    .5    .5]"  Multiplication=Matrix(K*u)
  Mux1 : Mux  Inputs=3
  dk : Outport
  qk : Outport  Port=2
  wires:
  K/1 -> Demux/1
  a/1 -> K/1
  Mux1/1 -> Fcn1/1, Fcn/1
  Fcn/1 -> dk/1
  Fcn1/1 -> qk/1
  th/1 -> Mux1/3
  Demux/1 -> Mux1/1
  Demux/2 -> Mux1/2

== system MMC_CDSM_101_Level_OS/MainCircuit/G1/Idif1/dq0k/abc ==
  dk : Inport
  qk : Inport  Port=2
  th : Inport  Port=3
  Fcn : Fcn  Expr=u(1)*cos(u(3)) - u(2)*sin(u(3))
  Fcn1 : Fcn  Expr=u(1)*sin(u(3)) + u(2)*cos(u(3))
  K : Gain  Gain="[1   0  1 ;  -.5   sqrt(3)/2    1 ;  -.5    -sqrt(3)/2    1]"  Multiplication=Matrix(K*u)
  Mux : Mux  Inputs=3
  Mux1 : Mux  Inputs=3
  a : Outport
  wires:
  th/1 -> Mux/3
  K/1 -> a/1
  Fcn1/1 -> Mux1/2
  Fcn/1 -> Mux1/1
  Mux1/1 -> K/1
  Mux/1 -> Fcn1/1, Fcn/1
  qk/1 -> Mux/2
  dk/1 -> Mux/1

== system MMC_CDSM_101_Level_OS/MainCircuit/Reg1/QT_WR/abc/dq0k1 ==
  a : Inport
  th : Inport  Port=2
  Demux : Demux  Outputs=3
  Fcn : Fcn  Expr=u(1)*cos(u(3)) + u(2)*sin(u(3))
  Fcn1 : Fcn  Expr=-u(1)*sin(u(3)) + u(2)*cos(u(3))
  K : Gain  Gain="2/3*[1   -.5   -.5;  0   sqrt(3)/2   -sqrt(3)/2;  .5    .5    .5]"  Multiplication=Matrix(K*u)
  Mux1 : Mux  Inputs=3
  dk : Outport
  qk : Outport  Port=2
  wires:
  K/1 -> Demux/1
  a/1 -> K/1
  Mux1/1 -> Fcn1/1, Fcn/1
  Fcn/1 -> dk/1
  Fcn1/1 -> qk/1
  th/1 -> Mux1/3
  Demux/1 -> Mux1/1
  Demux/2 -> Mux1/2

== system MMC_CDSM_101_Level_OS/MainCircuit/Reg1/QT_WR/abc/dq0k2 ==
  a : Inport
  th : Inport  Port=2
  Demux : Demux  Outputs=3
  Fcn : Fcn  Expr=u(1)*cos(u(3)) + u(2)*sin(u(3))
  Fcn1 : Fcn  Expr=-u(1)*sin(u(3)) + u(2)*cos(u(3))
  K : Gain  Gain="2/3*[1   -.5   -.5;  0   sqrt(3)/2   -sqrt(3)/2;  .5    .5    .5]"  Multiplication=Matrix(K*u)
  Mux1 : Mux  Inputs=3
  dk : Outport
  qk : Outport  Port=2
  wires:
  Demux/2 -> Mux1/2
  Demux/1 -> Mux1/1
  th/1 -> Mux1/3
  Fcn1/1 -> qk/1
  Fcn/1 -> dk/1
  Mux1/1 -> Fcn/1, Fcn1/1
  a/1 -> K/1
  K/1 -> Demux/1

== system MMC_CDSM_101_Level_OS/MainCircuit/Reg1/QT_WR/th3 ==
  abc : Inport
  C : ComplexToMagnitudeAngle
  Demux : Demux  Outputs=3
  K : Gain  Gain="2/3*[1   -.5   -.5;  0   sqrt(3)/2   -sqrt(3)/2;  .5    .5    .5]"  Multiplication=Matrix(K*u)
  R : RealImagToComplex
  |u| : Outport
  th : Outport  Port=2
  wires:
  C/1 -> |u|/1
  K/1 -> Demux/1
  abc/1 -> K/1
  Demux/1 -> R/1
  Demux/2 -> R/2
  R/1 -> C/1
  C/2 -> th/1

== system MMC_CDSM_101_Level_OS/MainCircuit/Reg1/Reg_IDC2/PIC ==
  c* : Inport  OutDataType=sfix(16)  OutScaling=2^0
  c : Inport  Port=2  OutDataType=sfix(16)  OutScaling=2^0
  Gain : Gain  Gain=Ki  ParameterDataType=sfix(16)  ParameterScaling=2^0  OutDataType=sfix(16)  OutScaling=2^0
  Gain1 : Gain  Gain=Kp  ParameterDataType=sfix(16)  ParameterScaling=2^0  OutDataType=sfix(16)  OutScaling=2^0
  Integrator : Integrator  UpperSaturationLimit=lim  LowerSaturationLimit=-lim
  Saturation : Saturate  UpperLimit=lim  LowerLimit=-lim
  Sum1 : Sum  Inputs=+-  OutDataType=sfix(16)  OutScaling=2^0
  Sum2 : Sum  OutDataType=sfix(16)  OutScaling=2^0
  e* : Outport  InitialOutput=0
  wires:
  Integrator/1 -> Sum2/2
  c*/1 -> Sum1/1
  c/1 -> Sum1/2
  Saturation/1 -> e*/1
  Sum2/1 -> Saturation/1
  Sum1/1 -> Gain1/1, Gain/1
  Gain1/1 -> Sum2/1
  Gain/1 -> Integrator/1

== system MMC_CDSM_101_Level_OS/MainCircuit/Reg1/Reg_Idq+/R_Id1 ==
  c* : Inport
  c : Inport  Port=2
  Gain : Gain  Gain=Ki
  Gain1 : Gain  Gain=Kp
  Integrator : Integrator  UpperSaturationLimit=lim  LowerSaturationLimit=-lim
  Saturation : Saturate  UpperLimit=lim  LowerLimit=-lim
  Sum1 : Sum  Inputs=+-
  Sum2 : Sum
  e* : Outport  InitialOutput=0
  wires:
  Gain/1 -> Integrator/1
  Gain1/1 -> Sum2/1
  Sum1/1 -> Gain/1, Gain1/1
  Sum2/1 -> Saturation/1
  Saturation/1 -> e*/1
  c/1 -> Sum1/2
  c*/1 -> Sum1/1
  Integrator/1 -> Sum2/2

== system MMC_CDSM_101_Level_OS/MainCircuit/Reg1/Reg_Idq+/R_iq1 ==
  c* : Inport
  c : Inport  Port=2
  Gain : Gain  Gain=Ki
  Gain1 : Gain  Gain=Kp
  Integrator : Integrator  UpperSaturationLimit=lim  LowerSaturationLimit=-lim
  Saturation : Saturate  UpperLimit=lim  LowerLimit=-lim
  Sum1 : Sum  Inputs=+-
  Sum2 : Sum
  e* : Outport  InitialOutput=0
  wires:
  Integrator/1 -> Sum2/2
  c*/1 -> Sum1/1
  c/1 -> Sum1/2
  Saturation/1 -> e*/1
  Sum2/1 -> Saturation/1
  Sum1/1 -> Gain1/1, Gain/1
  Gain1/1 -> Sum2/1
  Gain/1 -> Integrator/1

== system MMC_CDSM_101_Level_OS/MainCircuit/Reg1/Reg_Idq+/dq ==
  dk : Inport
  qk : Inport  Port=2
  0k : Inport  Port=3
  th : Inport  Port=4
  Fcn : Fcn  Expr=u(1)*cos(u(3)) - u(2)*sin(u(3))
  Fcn1 : Fcn  Expr=u(1)*sin(u(3)) + u(2)*cos(u(3))
  K : Gain  Gain="[1   0  1 ;  -.5   sqrt(3)/2    1 ;  -.5    -sqrt(3)/2    1]"  Multiplication=Matrix(K*u)
  Mux : Mux  Inputs=3
  Mux1 : Mux  Inputs=3
  a : Outport
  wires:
  dk/1 -> Mux/1
  qk/1 -> Mux/2
  Mux/1 -> Fcn/1, Fcn1/1
  K/1 -> a/1
  Mux1/1 -> K/1
  Fcn/1 -> Mux1/1
  Fcn1/1 -> Mux1/2
  th/1 -> Mux/3
  0k/1 -> Mux1/3
